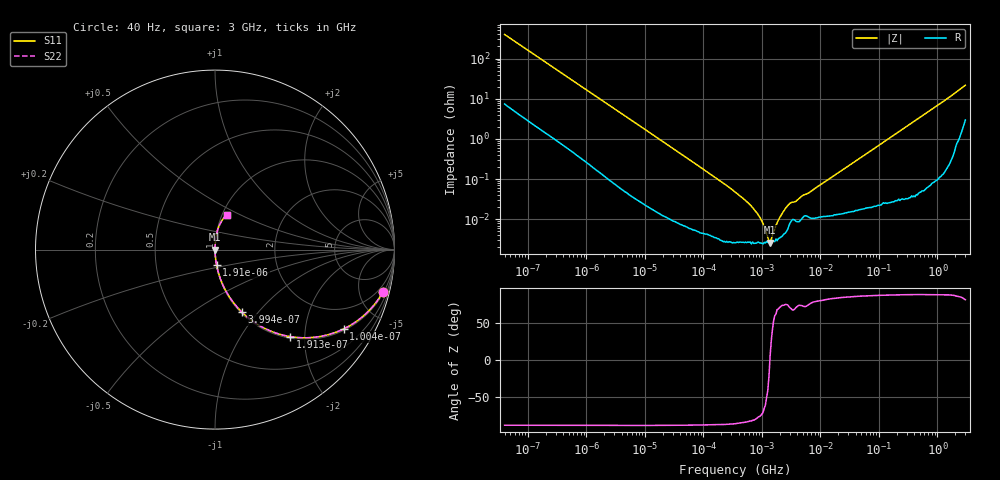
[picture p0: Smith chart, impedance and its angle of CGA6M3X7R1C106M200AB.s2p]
! S-parameter Generated by TDK Corporation
! Copyright(C) 2015 TDK Corporation.
! All Rights Reserved.
! TDK P/N: CGA6M3X7R1C106M200AB (Multilayer Ceramic Chip Capacitors)
! Property: C=10uF
! Size(LxWxT): 3.2x2.5x2mm, 0.126x0.098x0.079inches
! Model Type: s2p (Touchstone File Format Version 1.0)
! Frequency: DC=Yes Start=0.00004MHz Stop=3000MHz 396points Log-sweep
! Note: This model was converted from impedance.
! Model Generated on Jun. 23, 2015
! Hash(MD5):
! Port Assignments:
!  1 ---| |--- 2
! Applicable Conditions:
!  Temperature = 25 degC
!  DC Bias Voltage = 0 V
!  Small Signal Operation
! Terms and conditions regarding TDK Simulation Models
! (1)This simulation model is being provided solely for informational purposes. Please refer to the specifications of the products in terms of detailed characteristics of such products.
! (2)In no event shall TDK Corporation of any of its subsidiaries be liable for any loss or damage arising, directly or indirectly,
!  From any information contained in this simulation model, including, but not limited to loss or damages arising from any inaccuracies, omissions or errors in connection with such information.
! (3)Any and all copyrights on this simulation model are owned by TDK Corporation.
!  Duplication or redistribution of this simulation model without prior written permission from TDK Corporation is prohibited.
! (4)This simulation model is subject to any modification or change without any prior notice.
! (5)Neither TDK Corporation nor any of its subsidiaries shall make any warranty, express or implied,
!  Including but not limited to the correctness, implied warranties of merchantability and fitness for a particular purpose with respect to this simulation models.
! (6)The use of this simulation model shall be deemed to have consented to the terms and conditions hereof.
# MHz S MA R 50
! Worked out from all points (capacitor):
!   395 points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, 40 Hz to 3 GHz, reference 50 ohm
!   read as one part in series: C = 9.98 uF near 41.88 Hz
!   lowest |Z| = 2.65 mohm at 1.378 MHz (marker M1)
!   series resonance near 1.368 MHz, so ESL is about 1.4 nH
!   S11 on the Smith chart (normalised r, x): 40 Hz: 1.15, -7.94; 100.4 Hz: 1.06, -3.21; 191.3 Hz: 1.03, -1.70; 399.4 Hz: 1.01, -0.82; 1.91 kHz: 1.00, -0.18; 3 GHz: 1.06, +0.43
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4e-05  0.9654 -14.1  0.2432 74.9  0.2432 74.9  0.9654 -14.1
6.63624e-05  0.9181 -22.4  0.3804 66.6  0.3804 66.6  0.9181 -22.4
0.0001004175  0.842 -31.7  0.525 57.3  0.525 57.3  0.842 -31.7
0.0001912643  0.6417 -49.1  0.756 39.9  0.756 39.9  0.6417 -49.1
0.0003994232  0.3775 -66.8  0.9196 22.2  0.9196 22.2  0.3775 -66.8
0.000834128  0.1948 -77.9  0.9778 11.2  0.9778 11.2  0.1948 -77.9
0.001909884  0.08805 -84.1  0.9949 5.1  0.9949 5.1  0.08805 -84.1
0.01739424  0.009984 -88.6  0.9998 0.6  0.9998 0.6  0.009984 -88.6
0.3464102  0.000481 -86.9  1 0.0  1 0.0  0.000481 -86.9
0.6598043  0.0002134 -83.4  1 0.0  1 0.0  0.0002134 -83.4
0.9534872  0.0001027 -75.6  1 0.0  1 0.0  0.0001027 -75.6
1.37789  2.646e-05 4.8  1 -0.0  1 -0.0  2.646e-05 4.8
1.901634  9.418e-05 69.6  1 -0.0  1 -0.0  9.418e-05 69.6
2.506407  0.0001843 75.7  1 -0.0  1 -0.0  0.0001843 75.7
3.013016  0.0002497 71.2  0.9999 -0.0  0.9999 -0.0  0.0002497 71.2
3.792615  0.0002797 71.3  0.9999 -0.0  0.9999 -0.0  0.0002797 71.3
4.998775  0.0003925 73.6  0.9999 -0.0  0.9999 -0.0  0.0003925 73.6
7.22376  0.0005232 78.3  0.9999 -0.0  0.9999 -0.0  0.0005232 78.3
150.6385  0.01043 88.0  0.9997 -0.6  0.9997 -0.6  0.01043 88.0
906.6656  0.06169 85.6  0.9972 -3.5  0.9972 -3.5  0.06169 85.6
1893.418  0.1297 80.7  0.9874 -7.4  0.9874 -7.4  0.1297 80.7
3000  0.2061 70.4  0.9508 -11.8  0.9508 -11.8  0.2061 70.4
